FUNCTION_BLOCK PS_UnitModeManager
VAR_INPUT
	Execute 		: BOOL;
	eModeCommand 	: E_PMLUnitMode;
	ePMLState		: E_PMLState;
END_VAR
VAR_OUTPUT
	eModeStatus 	: E_PMLUnitMode;
	Done 			: BOOL;
	Error 			: BOOL;
	ErrorID 		: UDINT;
END_VAR
VAR
	fbTrigger		: R_TRIG;
END_VAR

fbTrigger(CLK := Execute);

IF fbTrigger.Q THEN (* rising edge Execute *)
	Done 		:= FALSE;
	Error 		:= FALSE;
	ErrorID 	:= 0;

     CASE eModeStatus OF
		E_PMLUnitMode.UNDEFINED:
					eModeStatus := eModeCommand;
					Done := TRUE;

		E_PMLUnitMode.AUTOMATIC:
					IF (ePMLState = E_PMLState.STOPPED) OR (ePMLState = E_PMLState.ABORTED) OR (ePMLState = E_PMLState.IDLE) THEN
						eModeStatus := eModeCommand;
						Done := TRUE;
					ELSIF ((ePMLState = E_PMLState.SUSPENDED) OR (ePMLState = E_PMLState.HELD) OR (ePMLState = E_PMLState.COMPLETE))
						AND (eModeCommand = E_PMLUnitMode.SEMIAUTOMATIC) THEN
		
						eModeStatus := eModeCommand;
						Done := TRUE;
					ELSIF (ePMLState = E_PMLState.HELD) AND (eModeCommand = E_PMLUnitMode.MAINTENANCE) THEN
						eModeStatus := eModeCommand;
						Done := TRUE;
					ELSE
						Error := TRUE;
						ErrorID := 1;
					END_IF

		E_PMLUnitMode.MAINTENANCE:
					IF (ePMLState = E_PMLState.STOPPED) OR (ePMLState = E_PMLState.ABORTED) OR (ePMLState = E_PMLState.IDLE) THEN
						eModeStatus := eModeCommand;
						Done := TRUE;
					ELSIF (ePMLState = E_PMLState.HELD) AND ((eModeCommand = E_PMLUnitMode.AUTOMATIC) OR (eModeCommand = E_PMLUnitMode.SEMIAUTOMATIC)) THEN
						eModeStatus := eModeCommand;
						Done := TRUE;
					ELSE
						Error := TRUE;
						ErrorID := 1;
					END_IF

		E_PMLUnitMode.MANUAL:
					IF (ePMLState = E_PMLState.STOPPED) OR (ePMLState = E_PMLState.ABORTED) OR (ePMLState = E_PMLState.IDLE) THEN
						eModeStatus := eModeCommand;
						Done := TRUE;
					ELSE
						Error := TRUE;
						ErrorID := 1;
					END_IF

		E_PMLUnitMode.SEMIAUTOMATIC:
					IF (ePMLState = E_PMLState.STOPPED) OR (ePMLState = E_PMLState.ABORTED) OR (ePMLState = E_PMLState.IDLE) THEN
						eModeStatus := eModeCommand;
						Done := TRUE;
					ELSIF ((ePMLState = E_PMLState.SUSPENDED) OR (ePMLState = E_PMLState.HELD) OR (ePMLState = E_PMLState.COMPLETE))
						AND (eModeCommand = E_PMLUnitMode.AUTOMATIC) THEN
		
						eModeStatus := eModeCommand;
						Done := TRUE;
					ELSIF (ePMLState = E_PMLState.HELD) AND (eModeCommand = E_PMLUnitMode.MAINTENANCE) THEN
						eModeStatus := eModeCommand;
						Done := TRUE;
					ELSE
						Error := TRUE;
						ErrorID := 1;
					END_IF

		E_PMLUnitMode.DRYRUN:
					eModeStatus := eModeCommand;
					Done 		:= TRUE;

		E_PMLUnitMode.USERMODE1:
					eModeStatus := eModeCommand;
					Done 		:= TRUE;

		E_PMLUnitMode.USERMODE2:
					eModeStatus := eModeCommand;
					Done 		:= TRUE;

		E_PMLUnitMode.IDLE:
					IF (ePMLState = E_PMLState.STOPPED) OR (ePMLState = E_PMLState.ABORTED) OR (ePMLState = E_PMLState.IDLE) THEN
						eModeStatus := eModeCommand;
						Done 		:= TRUE;
					ELSE
						Error 	:= TRUE;
						ErrorID := 1;
					END_IF

		E_PMLUnitMode.ESTOP:
					IF (ePMLState = E_PMLState.STOPPED) OR (ePMLState = E_PMLState.ABORTED) OR (ePMLState = E_PMLState.IDLE) THEN
						 eModeStatus := eModeCommand;
						 Done 		:= TRUE;
					ELSE
						 Error 	:= TRUE;
						 ErrorID := 1;
					END_IF
     END_CASE
END_IF

 (* reset with bExecute = FALSE *)
 IF NOT Execute THEN
     Done 		:= FALSE;
     Error 		:= FALSE;
     ErrorID 	:= 0;
 END_IF

END_FUNCTION_BLOCK
